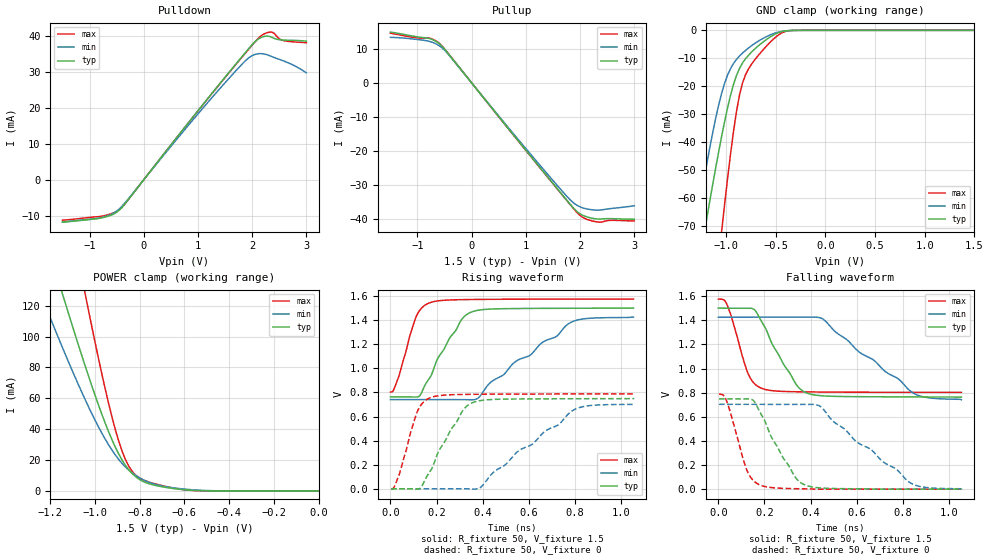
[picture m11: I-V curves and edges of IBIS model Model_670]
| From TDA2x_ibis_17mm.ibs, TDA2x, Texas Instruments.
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| Model based on original model for DDR_DIFFIOPB_V
|   Sub model SR100_DRV48_1P5
[model]   Model_670
|[Description]  [1.5V-I/O-X-X]
|   , ,
|[Input Load]
|[Output Drive]
|Voltage   1.5V
|Mode   I/O
Model_type   I/O
Polarity   Non-Inverting
Enable   Active-Low
Vinl =  0.65
Vinh =  0.85
Cref =  15.0000pF
Rref =  100.0000M
Vref =  0V
Vmeas =  0.75
C_comp   2p   2p   2p
[Model Spec]
Vinl   0.65   0.6125   0.6875
Vinh   0.85   0.8125   0.8875
[Receiver Thresholds]
Tslew_ac = 0.5n
Vth= 0.75
Vth_max= 0.7875
Vth_min= 0.675
Vinh_ac= 0.175
Vinh_dc= 0.1
Vinl_ac= -0.175
Vinl_dc= -0.1
[Temperature Range]   25   125   -40
[Voltage Range]   1.5   1.425   1.575
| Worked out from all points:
|   slope of the pulldown table from 0 to 0.225 V, typ, clamps not added: 51.5 ohm
|   slope of the pullup table from 0 to 0.225 V, typ, clamps not added: 50.1 ohm
|   GND clamp passes 1 mA (typ) near -0.48 V on its own axis
|   POWER clamp passes 1 mA (typ) near -0.62 V on its own axis
|   rising waveform, R_fixture 50, V_fixture 1.5: 20-80 % time 126ps typ, 301ps min, 69.5ps max; typ from 0.763 V to 1.5 V
|   rising waveform, R_fixture 50, V_fixture 0: 20-80 % time 125ps typ, 295ps min, 69.8ps max; typ from 0 V to 0.749 V
|   falling waveform, R_fixture 50, V_fixture 1.5: 20-80 % time 125ps typ, 281ps min, 71ps max; typ from 1.5 V to 0.763 V
|   falling waveform, R_fixture 50, V_fixture 0: 20-80 % time 126ps typ, 287ps min, 70.4ps max; typ from 0.749 V to 0 V
[POWER_clamp]
-1.5V     302.8mA    223.9mA    484.4mA
-1.242V   174.3mA    127.3mA    279.1mA
-1.136V   123.3mA    89.68mA    196.8mA
-1.045V   81.65mA    59.62mA    128.8mA
-1.03V    75mA       54.92mA    117.8mA
-939.4mV  38.44mA    29.91mA    56.84mA
-893.9mV  23.93mA    20.41mA    32.31mA
-848.5mV  13.61mA    13.43mA    15.91mA
-803mV    7.623mA    8.663mA    8.564mA
-712.1mV  3.022mA    3.561mA    3.877mA
-575.8mV  470.5uA    872uA      449uA
0V        112.6nA    435.6nA    613.8nA
[Pulldown]
-1.5V     -11.81mA   -11.79mA   -11.27mA
-727.3mV  -10.45mA   -10.3mA    -10mA
-545.5mV  -9.463mA   -9.189mA   -9.136mA
-409.1mV  -7.817mA   -7.49mA    -7.751mA
1.227V    23.47mA    22.31mA    23.4mA
1.818V    34.37mA    32.24mA    34.22mA
2V        37.61mA    34.55mA    37.45mA
2.136V    39.37mA    35.1mA     39.71mA
2.318V    39.9mA     34.55mA    41.07mA
2.409V    39.32mA    34mA       40.72mA
2.545V    38.91mA    33.26mA    38.88mA
3V        38.57mA    29.76mA    38.14mA
[Pullup]
-1.5V     14.98mA    13.43mA    14.66mA
-1V       13.57mA    12.78mA    13.25mA
-772.7mV  13.05mA    12.2mA     13.19mA
-590.9mV  11.46mA    10.89mA    11.59mA
-409.1mV  8.169mA    8.001mA    8.195mA
1.409V    -27.86mA   -27.07mA   -27.94mA
1.773V    -34.91mA   -33.72mA   -35mA
1.909V    -37.4mA    -35.72mA   -37.61mA
2.045V    -38.99mA   -36.82mA   -39.6mA
2.273V    -40.02mA   -37.48mA   -40.87mA
2.591V    -40.02mA   -37mA      -40.5mA
3V        -40.19mA   -36.21mA   -40.69mA
[GND_clamp]
-1.5V     -133.6mA   -115.7mA   -234.3mA
-1.288V   -87.29mA   -67.59mA   -156.8mA
-1.197V   -68.11mA   -48.64mA   -124.4mA
-1.045V   -38.25mA   -22.77mA   -72.51mA
-1.015V   -32.88mA   -19.1mA    -62.74mA
-954.5mV  -23.3mA    -13.72mA   -44.4mA
-863.6mV  -13.6mA    -9.192mA   -23.11mA
-803mV    -10.18mA   -7.193mA   -15.89mA
-681.8mV  -5.771mA   -4.027mA   -9.287mA
-500mV    -1.264mA   -914.7uA   -2.429mA
-348.5mV  -52.39uA   -75.11uA   -85.87uA
1.5V      112.6nA    528.1nA    514.5nA
[Ramp]
dV/dt_f 0.44251968/0.12525455n 0.41138958/0.28219457n 0.46379358/71.007829p
dV/dt_r 0.45069069/0.12510149n 0.42380059/0.29644022n  0.4737608/69.91952p
R_load = 50
[Rising Waveform]
R_fixture = 50
V_fixture = 1.5
V_fixture_min = 1.425
V_fixture_max = 1.575
0s        763.3mV    740.8mV    803.2mV
35.8ps    762.6mV    740.7mV    928.9mV
112ps     761.6mV    740.7mV    1.43V
167.2ps   911.3mV    740.8mV    1.542V
255.2ps   1.247V     740.4mV    1.567V
313.2ps   1.417V     740.3mV    1.57V
353.7ps   1.469V     738.8mV    1.572V
538.5ps   1.496V     1.051V     1.574V
781.4ps   1.499V     1.382V     1.575V
1.053ns   1.5V       1.425V     1.575V
[Rising Waveform]
R_fixture = 50
V_fixture = 0
V_fixture_min = 0
V_fixture_max = 0
3.237ps   0V         0V         0V
38.52ps   0V         0V         119.7mV
116.4ps   -2.411mV   0V         640.4mV
173.3ps   147.5mV    0V         756.4mV
211.1ps   319mV      0V         773.5mV
310.3ps   640.7mV    0V         783.2mV
361.1ps   719mV      -3.069mV   784.6mV
390.4ps   732.7mV    12.1mV     785.1mV
796.6ps   747.7mV    657.5mV    787.2mV
1.056ns   748.7mV    703.3mV    787.3mV
[Falling Waveform]
R_fixture = 50
V_fixture = 1.5
V_fixture_min = 1.425
V_fixture_max = 1.575
0s        1.5V       1.425V     1.575V
40.04ps   1.5V       1.425V     1.518V
133.6ps   1.501V     1.425V     938.2mV
159.1ps   1.482V     1.425V     869.7mV
190.5ps   1.379V     1.425V     833.6mV
334.3ps   876.1mV    1.425V     807.3mV
385.1ps   795.9mV    1.426V     805.9mV
455.3ps   772.7mV    1.407V     804.6mV
849.7ps   764.4mV    790.7mV    802.7mV
1.053ns   763.3mV    740.8mV    802.5mV
[Falling Waveform]
R_fixture = 50
V_fixture = 0
V_fixture_min = 0
V_fixture_max = 0
3.237ps   748.7mV    703.3mV    787.3mV
38.01ps   748.9mV    703.3mV    718.8mV
127.6ps   749mV      703.3mV    140.3mV
153.7ps   730.9mV    703.3mV    67.46mV
183.9ps   624.8mV    703.3mV    31.81mV
329.6ps   109.3mV    703.1mV    4.025mV
379.1ps   32mV       703.6mV    2.58mV
444ps     9.837mV    682.7mV    0V
835.1ps   0V         47.74mV    0V
1.056ns   0V         0V         0V
